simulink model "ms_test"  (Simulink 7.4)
settings: Solver=ode23t  StartTime=0.0  StopTime=9  RelTol=1e-5
undefined symbols (not defined in the file or in its folder): bits, D1, Delta
libraries: powerlib x25, powerlib_extras x3, dspswit3 x1

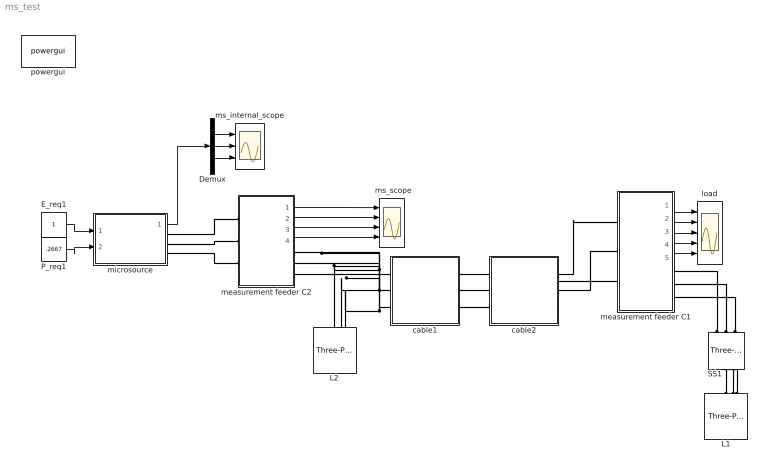
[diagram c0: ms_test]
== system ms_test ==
  " ms_scope" : Scope  NumInputPorts=4
  Demux : Demux  Outputs=3
  E_req1 : Constant  OutDataType=fixdt(1, 16)  OutScaling=2^0
  L1 : powerlib/Elements/Three-Phase Series RLC Load  DialogController=POWERSYS.PowerSysDialog  PhysicalDomain=powersysdomain  SubClassName=unknown  LeftPortType=p1  RightPortType=p1  LConnTagsString=A|B|C  Configuration=Y (grounded)  NominalVoltage=208  NominalFrequency=60  ActivePower=4000  InductivePower=0  CapacitivePower=0  Measurements=None
  L2 : powerlib/Elements/Three-Phase Series RLC Load  DialogController=POWERSYS.PowerSysDialog  PhysicalDomain=powersysdomain  SubClassName=unknown  LeftPortType=p1  RightPortType=p1  LConnTagsString=A|B|C  Configuration=Y (grounded)  NominalVoltage=208  NominalFrequency=60  ActivePower=1897  InductivePower=0  CapacitivePower=0  Measurements=None
  P_req1 : Constant  Value=.2667  OutDataType=fixdt(1, 16)  OutScaling=2^0
  SS1 : powerlib/Elements/Three-Phase Breaker  DialogController=POWERSYS.PowerSysDialog  SystemSampleTime=-1  InitialState=open  SwitchA=on  SwitchB=on  SwitchC=on  SwitchTimes=[1.7 7]  External=off  BreakerResistance=.001  SnubberResistance=1e6  SnubberCapacitance=inf  Measurements=None
  cable1 : Subsystem  mask{R=.002657, L=.000641, C=2020}
  cable2 : Subsystem  mask{R=0.0168, L=0.00407, C=336}
  load : Scope  NumInputPorts=5
  measurement feeder C1 : Subsystem
  measurement feeder C2 : Subsystem
  microsource : Subsystem  AncestorBlock=|
      | UWM_blocks/inverter-based
      | DG (simplified)
      | 208V - 15kVA
  ms_internal_scope : Scope  NumInputPorts=3
  powergui : powerlib/powergui  Priority=1  SystemSampleTime=-1  SimulationMode=Discrete  SampleTime=50e-6  frequency=60  SPID=off  DisableSnubberDevices=off  DisableRonSwitches=off  DisableVfSwitches=off  SwTol=0  Interpol=off  frequencyindice=0  echomessages=off  HookPort=off  DisplayEquations=off  FunctionMessages=off  EnableUseOfTLC=off  x0status=blocks  RestoreLinks=warning  Frange=[0:2:500]  Ylog=off  Xlog=on  ShowGrid=off  save=off  variable=ZData  ZoomFFT=on  StartTime=0.0  cycles=1  DisplayStyle=1  fundamental=60  FreqAxis=off  MaxFrequency=1000  frequencyindicesteady=1  RmsSteady=1  display=off  Ts=0  methode=off
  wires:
  measurement feeder C2/1(Vabc) -> " ms_scope"/1
  measurement feeder C2/2(Iabc) -> " ms_scope"/2
  measurement feeder C2/3(PQ) -> " ms_scope"/3
  measurement feeder C2/4(RMS (V-I)) -> " ms_scope"/4
  measurement feeder C1/5(w) -> load/5
  measurement feeder C1/4(RMS (V-I)) -> load/4
  measurement feeder C1/3(PQ) -> load/3
  measurement feeder C1/2(Iabc) -> load/2
  measurement feeder C1/1(Vabc) -> load/1
  P_req1/1 -> microsource/2(P_req)
  E_req1/1 -> microsource/1(E_req)
  Demux/2 -> ms_internal_scope/2
  Demux/1 -> ms_internal_scope/1
  Demux/3 -> ms_internal_scope/3
  microsource/1(m) -> Demux/1
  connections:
  cable1/RConn1 -- L2/LConn1 -- measurement feeder C2/RConn1
  cable1/RConn2 -- L2/LConn2 -- measurement feeder C2/RConn2
  cable1/RConn3 -- L2/LConn3 -- measurement feeder C2/RConn3
  microsource/RConn1 -- measurement feeder C2/LConn1
  microsource/RConn2 -- measurement feeder C2/LConn2
  microsource/RConn3 -- measurement feeder C2/LConn3
  L1/LConn1 -- SS1/RConn1
  L1/LConn2 -- SS1/RConn2
  L1/LConn3 -- SS1/RConn3
  SS1/LConn1 -- measurement feeder C1/RConn1
  SS1/LConn2 -- measurement feeder C1/RConn2
  SS1/LConn3 -- measurement feeder C1/RConn3
  cable2/LConn1 -- measurement feeder C1/LConn1
  cable2/LConn2 -- measurement feeder C1/LConn2
  cable2/LConn3 -- measurement feeder C1/LConn3
  cable1/LConn1 -- cable2/RConn1
  cable1/LConn2 -- cable2/RConn2
  cable1/LConn3 -- cable2/RConn3

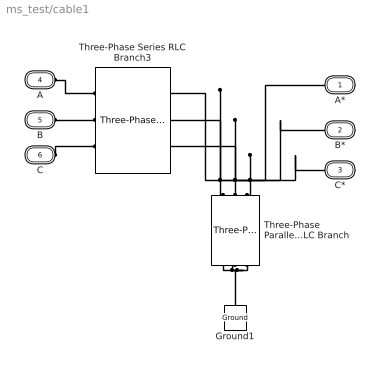
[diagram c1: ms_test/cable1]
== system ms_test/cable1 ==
  Ground1 : powerlib/Elements/Ground  DialogController=POWERSYS.PowerSysDialog  PhysicalDomain=powersysdomain  SubClassName=unknown  LeftPortType=p1  RightPortType=p1  LConnTagsString=a
  Three-Phase Parallel RLC Branch : powerlib/Elements/Three-Phase Parallel RLC Branch  DialogController=POWERSYS.PowerSysDialog  PhysicalDomain=powersysdomain  SubClassName=unknown  LeftPortType=p1  RightPortType=p1  LConnTagsString=A|B|C  RConnTagsString=A|B|C  BranchType=C  Resistance=1  Inductance=1e-3  Capacitance=1/(C*2*pi*60)  Measurements=None
  Three-Phase Series RLC Branch3 : powerlib/Elements/Three-Phase Series RLC Branch  DialogController=POWERSYS.PowerSysDialog  PhysicalDomain=powersysdomain  SubClassName=unknown  LeftPortType=p1  RightPortType=p1  LConnTagsString=A|B|C  RConnTagsString=A|B|C  BranchType=RL  Resistance=R  Inductance=L/(2*pi*60)  Capacitance=1/(336*2*pi*60)  Measurements=None
  A* : PMIOPort  Tag=PMCPort  Port=1  Side=Right
  B* : PMIOPort  Tag=PMCPort  Port=2  Side=Right
  C* : PMIOPort  Tag=PMCPort  Port=3  Side=Right
  A : PMIOPort  Tag=PMCPort  Port=4  Side=Left
  B : PMIOPort  Tag=PMCPort  Port=5  Side=Left
  C : PMIOPort  Tag=PMCPort  Port=6  Side=Left
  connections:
  Three-Phase Parallel RLC Branch/RConn3 -- Ground1/LConn1 -- Three-Phase Parallel RLC Branch/RConn2 -- Three-Phase Parallel RLC Branch/RConn1
  Three-Phase Parallel RLC Branch/LConn1 -- A*/RConn1 -- Three-Phase Series RLC Branch3/LConn1
  Three-Phase Parallel RLC Branch/LConn2 -- B*/RConn1 -- Three-Phase Series RLC Branch3/LConn2
  Three-Phase Parallel RLC Branch/LConn3 -- C*/RConn1 -- Three-Phase Series RLC Branch3/LConn3
  A/RConn1 -- Three-Phase Series RLC Branch3/RConn1
  B/RConn1 -- Three-Phase Series RLC Branch3/RConn2
  C/RConn1 -- Three-Phase Series RLC Branch3/RConn3

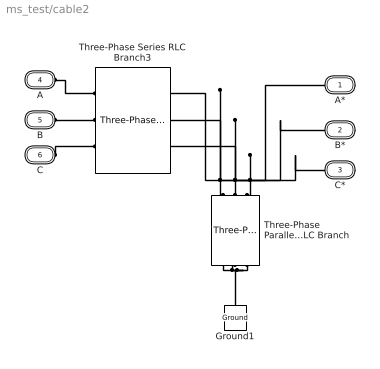
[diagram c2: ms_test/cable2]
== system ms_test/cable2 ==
  Ground1 : powerlib/Elements/Ground  DialogController=POWERSYS.PowerSysDialog  PhysicalDomain=powersysdomain  SubClassName=unknown  LeftPortType=p1  RightPortType=p1  LConnTagsString=a
  Three-Phase Parallel RLC Branch : powerlib/Elements/Three-Phase Parallel RLC Branch  DialogController=POWERSYS.PowerSysDialog  PhysicalDomain=powersysdomain  SubClassName=unknown  LeftPortType=p1  RightPortType=p1  LConnTagsString=A|B|C  RConnTagsString=A|B|C  BranchType=C  Resistance=1  Inductance=1e-3  Capacitance=1/(C*2*pi*60)  Measurements=None
  Three-Phase Series RLC Branch3 : powerlib/Elements/Three-Phase Series RLC Branch  DialogController=POWERSYS.PowerSysDialog  PhysicalDomain=powersysdomain  SubClassName=unknown  LeftPortType=p1  RightPortType=p1  LConnTagsString=A|B|C  RConnTagsString=A|B|C  BranchType=RL  Resistance=R  Inductance=L/(2*pi*60)  Capacitance=1/(336*2*pi*60)  Measurements=None
  A* : PMIOPort  Tag=PMCPort  Port=1  Side=Right
  B* : PMIOPort  Tag=PMCPort  Port=2  Side=Right
  C* : PMIOPort  Tag=PMCPort  Port=3  Side=Right
  A : PMIOPort  Tag=PMCPort  Port=4  Side=Left
  B : PMIOPort  Tag=PMCPort  Port=5  Side=Left
  C : PMIOPort  Tag=PMCPort  Port=6  Side=Left
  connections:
  Three-Phase Parallel RLC Branch/RConn3 -- Ground1/LConn1 -- Three-Phase Parallel RLC Branch/RConn2 -- Three-Phase Parallel RLC Branch/RConn1
  Three-Phase Parallel RLC Branch/LConn1 -- A*/RConn1 -- Three-Phase Series RLC Branch3/LConn1
  Three-Phase Parallel RLC Branch/LConn2 -- B*/RConn1 -- Three-Phase Series RLC Branch3/LConn2
  Three-Phase Parallel RLC Branch/LConn3 -- C*/RConn1 -- Three-Phase Series RLC Branch3/LConn3
  A/RConn1 -- Three-Phase Series RLC Branch3/RConn1
  B/RConn1 -- Three-Phase Series RLC Branch3/RConn2
  C/RConn1 -- Three-Phase Series RLC Branch3/RConn3

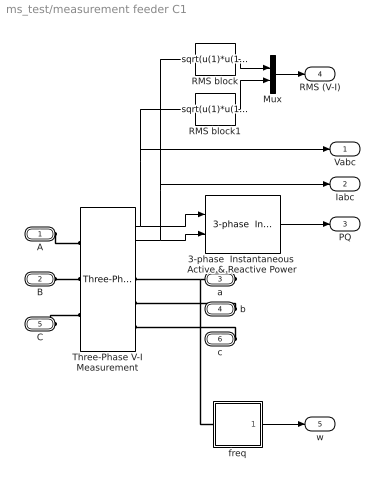
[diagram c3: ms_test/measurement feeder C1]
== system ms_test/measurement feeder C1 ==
  3-phase  Instantaneous  Active & Reactive Power : powerlib_extras/Measurements/3-phase  Instantaneous  Active & Reactive Power  DialogController=POWERSYS.PowerSysDialog  SystemSampleTime=-1
  Mux : Mux  Inputs=2
  RMS block : Fcn  Expr=sqrt(u(1)*u(1)+u(2)*u(2)+u(3)*u(3))/sqrt(3)
  RMS block1 : Fcn  Expr=sqrt(u(1)*u(1)+u(2)*u(2)+u(3)*u(3))/sqrt(3)
  Three-Phase V-I Measurement : powerlib/Measurements/Three-Phase V-I Measurement  DialogController=POWERSYS.PowerSysDialog  SystemSampleTime=-1  VoltageMeasurement=phase-to-ground  SetLabelV=off  LabelV=Vabc  Vpu=off  CurrentMeasurement=yes  SetLabelI=off  LabelI=Iabc  Ipu=off  Pbase=100e6  Vbase=500e3  OutputType=Complex  PhasorSimulation=off  PSBequivalent=0
  freq : Subsystem  AncestorBlock=|
      | UWM_blocks/frequency
      | measurement
      | (zero-crossings)
  A : PMIOPort  Port=1  Side=Left
  B : PMIOPort  Port=2  Side=Left
  a : PMIOPort  Port=3  Side=Right
  b : PMIOPort  Port=4  Side=Right
  C : PMIOPort  Port=5  Side=Left
  c : PMIOPort  Port=6  Side=Right
  Vabc : Outport  OutDataType=fixdt(1, 16)  OutScaling=2^0
  Iabc : Outport  Port=2  OutDataType=fixdt(1, 16)  OutScaling=2^0
  PQ : Outport  Port=3  OutDataType=fixdt(1, 16)  OutScaling=2^0
  RMS (V-I) : Outport  Port=4  OutDataType=fixdt(1, 16)  OutScaling=2^0
  w : Outport  Port=5  OutDataType=fixdt(1, 16)  OutScaling=2^0
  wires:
  Three-Phase V-I Measurement/1 -> Vabc/1, RMS block1/1, 3-phase  Instantaneous  Active & Reactive Power/1
  Three-Phase V-I Measurement/2 -> Iabc/1, RMS block/1, 3-phase  Instantaneous  Active & Reactive Power/2
  Mux/1 -> RMS (V-I)/1
  RMS block/1 -> Mux/1
  RMS block1/1 -> Mux/2
  3-phase  Instantaneous  Active & Reactive Power/1 -> PQ/1
  freq/1(w (Hz)) -> w/1
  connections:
  c/RConn1 -- Three-Phase V-I Measurement/RConn3
  C/RConn1 -- Three-Phase V-I Measurement/LConn3
  b/RConn1 -- Three-Phase V-I Measurement/RConn2
  a/RConn1 -- Three-Phase V-I Measurement/RConn1 -- freq/LConn1
  B/RConn1 -- Three-Phase V-I Measurement/LConn2
  A/RConn1 -- Three-Phase V-I Measurement/LConn1

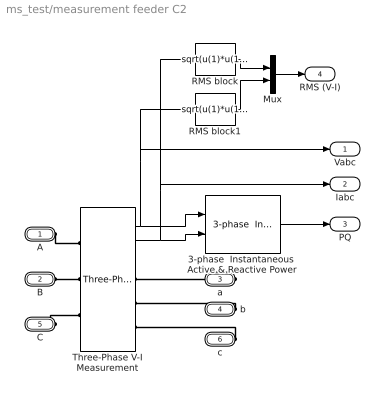
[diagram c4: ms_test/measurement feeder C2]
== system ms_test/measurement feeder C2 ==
  3-phase  Instantaneous  Active & Reactive Power : powerlib_extras/Measurements/3-phase  Instantaneous  Active & Reactive Power  DialogController=POWERSYS.PowerSysDialog  SystemSampleTime=-1
  Mux : Mux  Inputs=2
  RMS block : Fcn  Expr=sqrt(u(1)*u(1)+u(2)*u(2)+u(3)*u(3))/sqrt(3)
  RMS block1 : Fcn  Expr=sqrt(u(1)*u(1)+u(2)*u(2)+u(3)*u(3))/sqrt(3)
  Three-Phase V-I Measurement : powerlib/Measurements/Three-Phase V-I Measurement  DialogController=POWERSYS.PowerSysDialog  SystemSampleTime=-1  VoltageMeasurement=phase-to-ground  SetLabelV=off  LabelV=Vabc  Vpu=off  CurrentMeasurement=yes  SetLabelI=off  LabelI=Iabc  Ipu=off  Pbase=100e6  Vbase=500e3  OutputType=Complex  PhasorSimulation=off  PSBequivalent=0
  A : PMIOPort  Port=1  Side=Left
  B : PMIOPort  Port=2  Side=Left
  a : PMIOPort  Port=3  Side=Right
  b : PMIOPort  Port=4  Side=Right
  C : PMIOPort  Port=5  Side=Left
  c : PMIOPort  Port=6  Side=Right
  Vabc : Outport  OutDataType=fixdt(1, 16)  OutScaling=2^0
  Iabc : Outport  Port=2  OutDataType=fixdt(1, 16)  OutScaling=2^0
  PQ : Outport  Port=3  OutDataType=fixdt(1, 16)  OutScaling=2^0
  RMS (V-I) : Outport  Port=4  OutDataType=fixdt(1, 16)  OutScaling=2^0
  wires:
  Three-Phase V-I Measurement/1 -> Vabc/1, RMS block1/1, 3-phase  Instantaneous  Active & Reactive Power/1
  Three-Phase V-I Measurement/2 -> Iabc/1, RMS block/1, 3-phase  Instantaneous  Active & Reactive Power/2
  Mux/1 -> RMS (V-I)/1
  RMS block/1 -> Mux/1
  RMS block1/1 -> Mux/2
  3-phase  Instantaneous  Active & Reactive Power/1 -> PQ/1
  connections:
  c/RConn1 -- Three-Phase V-I Measurement/RConn3
  C/RConn1 -- Three-Phase V-I Measurement/LConn3
  b/RConn1 -- Three-Phase V-I Measurement/RConn2
  a/RConn1 -- Three-Phase V-I Measurement/RConn1
  B/RConn1 -- Three-Phase V-I Measurement/LConn2
  A/RConn1 -- Three-Phase V-I Measurement/LConn1

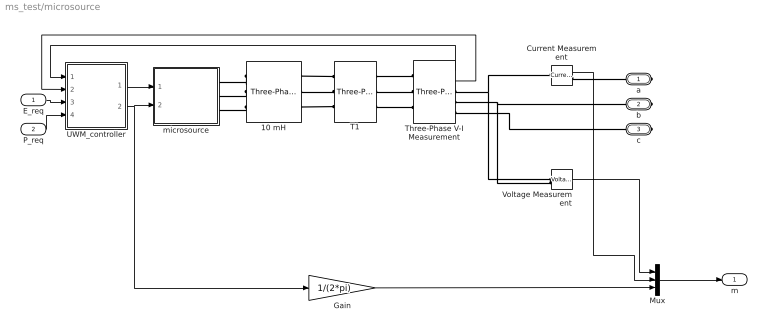
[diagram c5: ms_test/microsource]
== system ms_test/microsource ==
  E_req : Inport
  P_req : Inport  Port=2
  10 mH : powerlib/Elements/Three-Phase Series RLC Branch  DialogController=POWERSYS.PowerSysDialog  PhysicalDomain=powersysdomain  SubClassName=unknown  LeftPortType=p1  RightPortType=p1  LConnTagsString=A|B|C  RConnTagsString=A|B|C  BranchType=L  Resistance=.0028  Inductance=5e-3  Capacitance=1e-6  Measurements=None
  Current Measurement : powerlib/Measurements/Current Measurement  DialogController=POWERSYS.PowerSysDialog  SystemSampleTime=-1  PhasorSimulation=off  OutputType=Complex  PSBequivalent=0
  Gain : Gain  Gain=1/(2*pi)  ParameterDataType=fixdt(1, 16)  ParameterScaling=2^0  OutDataType=fixdt(1, 16)  OutScaling=2^0
  Mux : Mux  Inputs=3
  T1 : powerlib/Elements/Three-Phase Transformer (Two Windings)  DialogController=POWERSYS.PowerSysDialog  SystemSampleTime=-1  Winding1Connection=Delta (D1)  UNITS=SI  NominalPower=[ 45e3 , 60 ]  Winding1=[208 0.02688 0.1075/(2*pi*60)]  Winding2Connection=Yg  Winding2=[208 0.005047 .0201/(2*pi*60)]  SetSaturation=off  Rm=100.e6  Lm=7650.8  Saturation=[0 0;1359.8 0.93633;5.6659e+05 1.186]  Hysteresis=off  DataFile='hysteresis'  SetInitialFlux=off  InitialFluxes=[0.62422 -0.62422 0.54618]  Measurements=None  MoreParameters=off  BreakLoop=off  DataType=on  TransfoNumber=1
  Three-Phase V-I Measurement : powerlib/Measurements/Three-Phase V-I Measurement  DialogController=POWERSYS.PowerSysDialog  SystemSampleTime=-1  VoltageMeasurement=phase-to-ground  SetLabelV=off  LabelV=Vabc  Vpu=off  CurrentMeasurement=yes  SetLabelI=off  LabelI=Iabc  Ipu=off  Pbase=100e6  Vbase=500e3  OutputType=Complex  PhasorSimulation=off  PSBequivalent=0
  UWM_controller : Subsystem  mask{Vbase=208, Sbase=15000}
  Voltage Measurement : powerlib/Measurements/Voltage Measurement  DialogController=POWERSYS.PowerSysDialog  SystemSampleTime=-1  PhasorSimulation=off  OutputType=Complex  PSBequivalent=0
  microsource : Subsystem
  a : PMIOPort  Port=1  Side=Right
  b : PMIOPort  Port=2  Side=Right
  c : PMIOPort  Port=3  Side=Right
  m : Outport  OutDataType=fixdt(1, 16)  OutScaling=2^0
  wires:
  E_req/1 -> UWM_controller/3(E_req)
  P_req/1 -> UWM_controller/4(P_req)
  Three-Phase V-I Measurement/1 -> UWM_controller/1(v_meas)
  Three-Phase V-I Measurement/2 -> UWM_controller/2(i_meas)
  UWM_controller/1(Vpk) -> microsource/1(Vpk)
  UWM_controller/2(w) -> microsource/2(w), Gain/1
  Mux/1 -> m/1
  Voltage Measurement/1 -> Mux/1
  Current Measurement/1 -> Mux/2
  Gain/1 -> Mux/3
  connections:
  Three-Phase V-I Measurement/RConn2 -- b/RConn1 -- Voltage Measurement/LConn2
  Three-Phase V-I Measurement/RConn3 -- c/RConn1
  Current Measurement/RConn1 -- a/RConn1
  Three-Phase V-I Measurement/RConn1 -- Current Measurement/LConn1 -- Voltage Measurement/LConn1
  10 mH/LConn2 -- microsource/RConn2
  10 mH/LConn1 -- microsource/RConn1
  10 mH/LConn3 -- microsource/RConn3
  T1/LConn1 -- 10 mH/RConn1
  T1/LConn2 -- 10 mH/RConn2
  T1/LConn3 -- 10 mH/RConn3
  T1/RConn1 -- Three-Phase V-I Measurement/LConn1
  T1/RConn2 -- Three-Phase V-I Measurement/LConn2
  T1/RConn3 -- Three-Phase V-I Measurement/LConn3

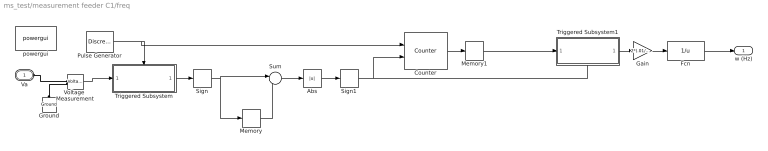
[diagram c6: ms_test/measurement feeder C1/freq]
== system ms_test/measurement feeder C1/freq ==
  Abs : Abs  OutDataType=fixdt(1, 16)  OutScaling=2^0
  Counter : dspswit3/Counter  Direction=Up  CountEvent=Rising edge  CounterSize=32 bits  MaxCount=255  InitialCount=0  Output=Count  HitValue=32  ResetInput=on  SamplesPerFrame=1  Ts=1  CntDtype=double  HitDtype=Logical
  Fcn : Fcn  Expr=1/u
  Gain : Gain  Gain=2*(.01/60)  ParameterDataType=fixdt(1, 16)  ParameterScaling=2^0  OutDataType=fixdt(1, 16)  OutScaling=2^0
  Ground : powerlib/Elements/Ground  DialogController=POWERSYS.PowerSysDialog  PhysicalDomain=powersysdomain  SubClassName=unknown  LeftPortType=p1  RightPortType=p1  LConnTagsString=a
  Memory : Memory
  Memory1 : Memory  InheritSampleTime=on
  Pulse Generator : DiscretePulseGenerator  PulseType=Time based  Amplitude=1  Period=.01/60  PulseWidth=50  PhaseDelay=0  SampleTime=1
  Sign : Signum
  Sign1 : Signum
  Sum : Sum  Inputs=|+-  OutDataType=fixdt(1, 16)  OutScaling=2^0
  Triggered Subsystem : Subsystem  TreatAsAtomicUnit=on
  Triggered Subsystem1 : Subsystem  TreatAsAtomicUnit=on
  Voltage  Measurement : powerlib/Measurements/Voltage Measurement  DialogController=POWERSYS.PowerSysDialog  SystemSampleTime=-1  PhasorSimulation=off  OutputType=Complex  PSBequivalent=0
  powergui : powerlib/powergui  Priority=1  SystemSampleTime=-1  SimulationMode=Continuous  SampleTime=50e-6  frequency=60  SPID=off  DisableSnubberDevices=off  DisableRonSwitches=off  DisableVfSwitches=off  SwTol=0  Interpol=off  frequencyindice=0  echomessages=off  HookPort=off  DisplayEquations=off  FunctionMessages=off  EnableUseOfTLC=off  x0status=blocks  RestoreLinks=warning  Frange=[0:2:500]  Ylog=off  Xlog=on  ShowGrid=off  save=off  variable=ZData  ZoomFFT=on  StartTime=0.0  cycles=1  DisplayStyle=1  fundamental=60  FreqAxis=off  MaxFrequency=1000  frequencyindicesteady=1  RmsSteady=1  display=off  Ts=0  methode=off
  Va : PMIOPort  Tag=PMCPort  Port=1  Side=Left
  w (Hz) : Outport
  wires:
  Pulse Generator/1 -> Triggered Subsystem/Trigger, Counter/1
  Triggered Subsystem/1(Out1) -> Sign/1
  Sign/1 -> Sum/1, Memory/1
  Memory/1 -> Sum/2
  Sum/1 -> Abs/1
  Abs/1 -> Sign1/1
  Sign1/1 -> Counter/2, Triggered Subsystem1/Trigger
  Triggered Subsystem1/1(Out1) -> Gain/1
  Gain/1 -> Fcn/1
  Counter/1 -> Memory1/1
  Memory1/1 -> Triggered Subsystem1/1(In1)
  Voltage  Measurement/1 -> Triggered Subsystem/1(In1)
  Fcn/1 -> w (Hz)/1
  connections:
  Ground/LConn1 -- Voltage  Measurement/LConn2
  Va/RConn1 -- Voltage  Measurement/LConn1

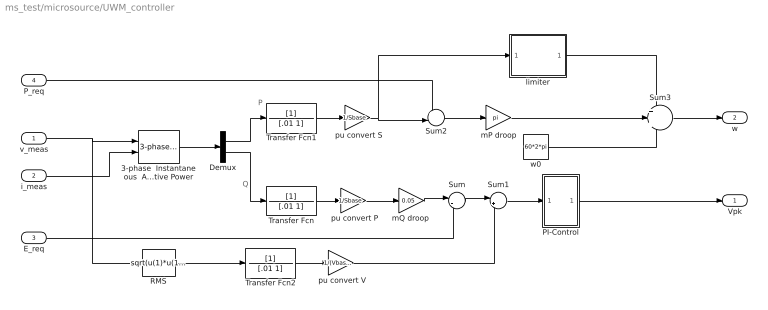
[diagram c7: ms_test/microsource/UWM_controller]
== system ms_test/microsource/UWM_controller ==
  note: P
  note: Q
  v_meas : Inport
  i_meas : Inport  Port=2
  E_req : Inport  Port=3
  P_req : Inport  Port=4
  " pu convert P" : Gain  Gain=1/Sbase  ParameterDataType=sfix(16)  ParameterScaling=2^0  OutDataType=sfix(16)  OutScaling=2^0
  " pu convert S" : Gain  Gain=1/Sbase  ParameterDataType=sfix(16)  ParameterScaling=2^0  OutDataType=sfix(16)  OutScaling=2^0
  " pu convert V" : Gain  Gain=1/(Vbase/sqrt(3))  ParameterDataType=sfix(16)  ParameterScaling=2^0  OutDataType=sfix(16)  OutScaling=2^0
  3-phase  Instantaneous  Active & Reactive Power : powerlib_extras/Measurements/3-phase  Instantaneous  Active & Reactive Power  DialogController=POWERSYS.PowerSysDialog  SystemSampleTime=-1
  Demux : Demux  Outputs=2
  PI-Control : Subsystem
  RMS : Fcn  Expr=sqrt(u(1)*u(1)+u(2)*u(2)+u(3)*u(3))/sqrt(3)
  Sum : Sum  Inputs=|-+  OutDataType=sfix(16)  OutScaling=2^0
  Sum1 : Sum  Inputs=|+-  OutDataType=sfix(16)  OutScaling=2^0
  Sum2 : Sum  Inputs=+-|  OutDataType=sfix(16)  OutScaling=2^0
  Sum3 : Sum  Inputs=+++  OutDataType=sfix(16)  OutScaling=2^0
  Transfer Fcn : TransferFcn  Denominator=[.01 1]
  Transfer Fcn1 : TransferFcn  Denominator=[.01 1]
  Transfer Fcn2 : TransferFcn  Denominator=[.01 1]
  limiter : Subsystem
  mP droop : Gain  Gain=pi  ParameterDataType=sfix(16)  ParameterScaling=2^0  OutDataType=sfix(16)  OutScaling=2^0
  "mQ droop " : Gain  Gain=0.05  ParameterDataType=sfix(16)  ParameterScaling=2^0  OutDataType=sfix(16)  OutScaling=2^0
  w0 : Constant  Value=60*2*pi  OutDataType=fixdt(1, 16)  OutScaling=2^0
  Vpk : Outport
  w : Outport  Port=2
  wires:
  Transfer Fcn2/1 -> " pu convert V"/1
  Transfer Fcn/1 -> " pu convert P"/1
  " pu convert P"/1 -> "mQ droop "/1
  Transfer Fcn1/1 -> " pu convert S"/1
  " pu convert S"/1 -> limiter/1(In1), Sum2/2
  i_meas/1 -> 3-phase  Instantaneous  Active & Reactive Power/2
  P_req/1 -> Sum2/1
  mP droop/1 -> Sum3/2
  limiter/1(Out1) -> Sum3/1
  w0/1 -> Sum3/3
  Sum2/1 -> mP droop/1
  Sum1/1 -> PI-Control/1(In1)
  Sum/1 -> Sum1/1
  "mQ droop "/1 -> Sum/1
  RMS/1 -> Transfer Fcn2/1
  Demux/2 -> Transfer Fcn/1
  Demux/1 -> Transfer Fcn1/1
  3-phase  Instantaneous  Active & Reactive Power/1 -> Demux/1
  v_meas/1 -> RMS/1, 3-phase  Instantaneous  Active & Reactive Power/1
  PI-Control/1(Out1) -> Vpk/1
  Sum3/1 -> w/1
  E_req/1 -> Sum/2
  " pu convert V"/1 -> Sum1/2

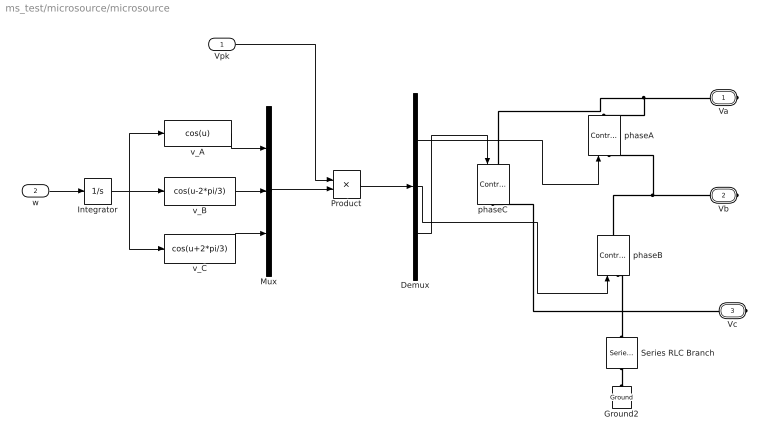
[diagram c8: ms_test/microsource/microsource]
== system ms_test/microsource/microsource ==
  Vpk : Inport  OutDataType=fixdt(1, 16)  OutScaling=2^0
  w : Inport  Port=2  OutDataType=fixdt(1, 16)  OutScaling=2^0
  Demux : Demux  Outputs=3
  Ground2 : powerlib/Elements/Ground  DialogController=POWERSYS.PowerSysDialog  PhysicalDomain=powersysdomain  SubClassName=unknown  LeftPortType=p1  RightPortType=p1  LConnTagsString=a
  Integrator : Integrator
  Mux : Mux  Inputs=3
  Product : Product  OutDataType=sfix(16)  OutScaling=2^0
  Series RLC Branch : powerlib/Elements/Series RLC Branch  DialogController=POWERSYS.PowerSysDialog  PhysicalDomain=powersysdomain  SubClassName=unknown  LeftPortType=p1  RightPortType=p1  LConnTagsString=__new0  RConnTagsString=__new0  BranchType=C  Resistance=1  Inductance=1e-3  SetiL0=off  InitialCurrent=0  Capacitance=1e-8  Setx0=off  InitialVoltage=0  Measurements=None
  phaseA : powerlib/Electrical Sources/Controlled Voltage Source  DialogController=POWERSYS.PowerSysDialog  SystemSampleTime=-1  Initialize=on  Source_Type=AC  Amplitude=0  Phase=0  Frequency=0  Measurements=None
  phaseB : powerlib/Electrical Sources/Controlled Voltage Source  DialogController=POWERSYS.PowerSysDialog  SystemSampleTime=-1  Initialize=on  Source_Type=AC  Amplitude=0  Phase=0  Frequency=0  Measurements=None
  phaseC : powerlib/Electrical Sources/Controlled Voltage Source  DialogController=POWERSYS.PowerSysDialog  SystemSampleTime=-1  Initialize=on  Source_Type=AC  Amplitude=0  Phase=0  Frequency=0  Measurements=None
  v_A : Fcn  Expr=cos(u)
  v_B : Fcn  Expr=cos(u-2*pi/3)
  v_C : Fcn  Expr=cos(u+2*pi/3)
  Va : PMIOPort  Tag=PMCPort  Port=1  Side=Right
  Vb : PMIOPort  Tag=PMCPort  Port=2  Side=Right
  Vc : PMIOPort  Tag=PMCPort  Port=3  Side=Right
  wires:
  Product/1 -> Demux/1
  Vpk/1 -> Product/1
  Mux/1 -> Product/2
  w/1 -> Integrator/1
  Integrator/1 -> v_A/1, v_B/1, v_C/1
  v_A/1 -> Mux/1
  v_B/1 -> Mux/2
  v_C/1 -> Mux/3
  Demux/1 -> phaseA/1
  Demux/2 -> phaseB/1
  Demux/3 -> phaseC/1
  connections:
  Vb/RConn1 -- phaseB/RConn1 -- phaseA/LConn1
  Va/RConn1 -- phaseC/LConn1 -- phaseA/RConn1
  Vc/RConn1 -- phaseC/RConn1
  Series RLC Branch/RConn1 -- Ground2/LConn1
  Series RLC Branch/LConn1 -- phaseB/LConn1

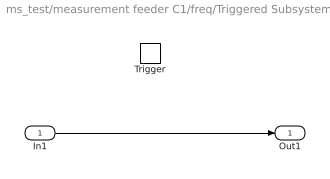
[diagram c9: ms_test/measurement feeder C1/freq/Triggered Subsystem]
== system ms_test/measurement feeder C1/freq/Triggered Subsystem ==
  In1 : Inport  OutDataType=fixdt(1, 16)  OutScaling=2^0
  Trigger : TriggerPort
  Out1 : Outport  OutDataType=fixdt(1, 16)  OutScaling=2^0
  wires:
  In1/1 -> Out1/1

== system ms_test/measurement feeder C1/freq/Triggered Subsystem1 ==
  In1 : Inport  OutDataType=fixdt(1, 16)  OutScaling=2^0
  Trigger : TriggerPort
  Out1 : Outport  OutDataType=fixdt(1, 16)  OutScaling=2^0
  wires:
  In1/1 -> Out1/1

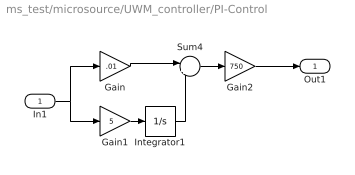
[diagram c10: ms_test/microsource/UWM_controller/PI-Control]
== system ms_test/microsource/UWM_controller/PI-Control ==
  In1 : Inport
  Gain : Gain  Gain=.01  ParameterDataType=sfix(16)  ParameterScaling=2^0  OutDataType=sfix(16)  OutScaling=2^0
  Gain1 : Gain  Gain=5  ParameterDataType=sfix(16)  ParameterScaling=2^0  OutDataType=sfix(16)  OutScaling=2^0
  Gain2 : Gain  Gain=750  ParameterDataType=sfix(16)  ParameterScaling=2^0  OutDataType=sfix(16)  OutScaling=2^0
  Integrator1 : Integrator  LimitOutput=on  UpperSaturationLimit=100  LowerSaturationLimit=-100  ZeroCross=off
  Sum4 : Sum  Inputs=|++  OutDataType=sfix(16)  OutScaling=2^0
  Out1 : Outport
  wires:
  Gain/1 -> Sum4/1
  Integrator1/1 -> Sum4/2
  In1/1 -> Gain1/1, Gain/1
  Gain1/1 -> Integrator1/1
  Sum4/1 -> Gain2/1
  Gain2/1 -> Out1/1

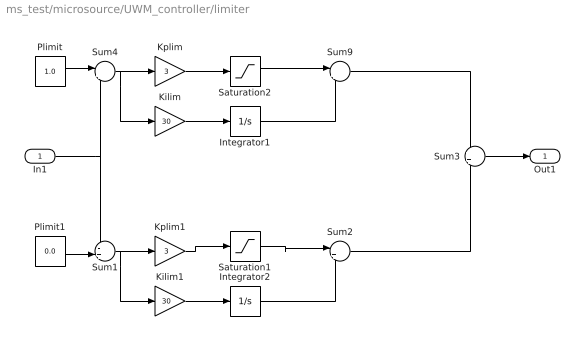
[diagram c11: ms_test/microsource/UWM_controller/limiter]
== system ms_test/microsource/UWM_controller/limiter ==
  In1 : Inport
  Integrator1 : Integrator  LimitOutput=on  UpperSaturationLimit=0  LowerSaturationLimit=-pi  ZeroCross=off
  Integrator2 : Integrator  LimitOutput=on  UpperSaturationLimit=pi  LowerSaturationLimit=0  ZeroCross=off
  Kilim : Gain  Gain=30  ParameterDataType=sfix(16)  ParameterScaling=2^0  OutDataType=sfix(16)  OutScaling=2^0
  Kilim1 : Gain  Gain=30  ParameterDataType=sfix(16)  ParameterScaling=2^0  OutDataType=sfix(16)  OutScaling=2^0
  Kplim : Gain  Gain=3  ParameterDataType=sfix(16)  ParameterScaling=2^0  OutDataType=sfix(16)  OutScaling=2^0
  Kplim1 : Gain  Gain=3  ParameterDataType=sfix(16)  ParameterScaling=2^0  OutDataType=sfix(16)  OutScaling=2^0
  Plimit : Constant  Value=1.0  OutDataType=sfix(16)  OutScaling=2^0
  Plimit1 : Constant  Value=0.0  OutDataType=sfix(16)  OutScaling=2^0
  Saturation1 : Saturate  UpperLimit=pi  LowerLimit=0  OutDataType=fixdt(1, 16)  OutScaling=2^0
  Saturation2 : Saturate  UpperLimit=0  LowerLimit=-pi  OutDataType=fixdt(1, 16)  OutScaling=2^0
  Sum1 : Sum  Inputs=-+|  OutDataType=sfix(16)  OutScaling=2^0
  Sum2 : Sum  Inputs=|++  OutDataType=sfix(16)  OutScaling=2^0
  Sum3 : Sum  OutDataType=sfix(16)  OutScaling=2^0
  Sum4 : Sum  Inputs=|+-  OutDataType=sfix(16)  OutScaling=2^0
  Sum9 : Sum  Inputs=|++  OutDataType=sfix(16)  OutScaling=2^0
  Out1 : Outport
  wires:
  Sum3/1 -> Out1/1
  Plimit1/1 -> Sum1/2
  Integrator2/1 -> Sum2/2
  Kilim1/1 -> Integrator2/1
  Sum1/1 -> Kilim1/1, Kplim1/1
  In1/1 -> Sum1/1, Sum4/2
  Integrator1/1 -> Sum9/2
  Kilim/1 -> Integrator1/1
  Sum4/1 -> Kilim/1, Kplim/1
  Plimit/1 -> Sum4/1
  Kplim1/1 -> Saturation1/1
  Saturation1/1 -> Sum2/1
  Kplim/1 -> Saturation2/1
  Saturation2/1 -> Sum9/1
  Sum9/1 -> Sum3/1
  Sum2/1 -> Sum3/2
